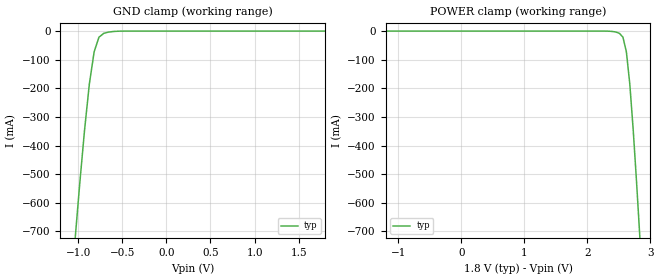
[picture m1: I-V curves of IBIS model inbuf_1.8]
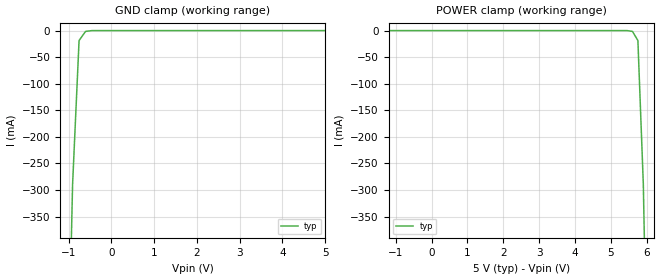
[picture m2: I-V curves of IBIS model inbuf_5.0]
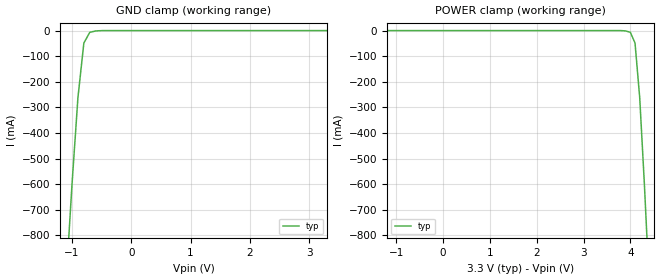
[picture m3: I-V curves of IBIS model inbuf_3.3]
|Texas Instruments Incorporated
|tmux2821, 2 Data Lane 1:1 15V Precision mux
[IBIS Ver]   4.1
[File name]   tmux2821.ibs
[Date]   04/10/25
[File Rev]   1.0
[Source]
| Texas Instruments Incorporated.
| ASC-INT-MPD
| 12500 TI Blvd
| Dallas, TX - 75243
[Notes]   Revision History:
| Rev 1.0: 04/10/25
| - Initial version of the model
| - Model generated from simulations in SPECTRE
| - C_comp although listed in numerical order of value are
|   obtained from varying PVT conditions. For PVT conditions for
|   each specific value refer the buffer description under
|   respective [Model]. IBIS model user is responsible for using
|   appropriate C_comp to simulate for Signal Integrity.
[Disclaimer]
| This model is designed as an aid for customers of Texas Instruments.
| TI and its licensors and suppliers make no warranties, either expressed
| or implied, with respect to this  model, including the warranties of
| merchantability or fitness for a particular purpose. The model is
| provided solely on an "as is" basis. The entire risk as to its quality
| and performance is with the customer.
| This model is subject to change without notice. Texas Instruments
| Incorporated is not responsible for updating this model.
[Copyright]
(C) Copyright 2025 Texas Instruments Incorporated.All rights reserved.
|  Component TMUX2821DSG 8-pin - DSG package
|  Part # TMUX2821DSG
[Component]   TMUX2821DSG
[Manufacturer]  TI
[Package]
|   typ   min   max
R_pkg   0.027   NA   NA
L_pkg   2.1992nH   NA   NA
C_pkg   0.2884pF   NA   NA
[Pin]   signal_name   model_name
   1   S1   sterm_fs_dual_7.5
   2   D1   dterm_fs_dual_7.5
   3   SEL2   inbuf
   4   GND   gnd
   5   S2   sterm_fs_dual_7.5
   6   D2   dterm_fs_dual_7.5
   7   SEL1   inbuf
   8   VDD   power
[Series Switch Groups]
On 1 /
On 2 /
Off 1 2 /
[Series Pin Mapping]  pin_2 model_name function_table_group
   1   2   switch_dual_7.5   1
   5   6   switch_dual_7.5   2
|  Component TMUX2821DDF 8-pin - DDF package
|  Part # TMUX2821DDF
[Component]   TMUX2821DDF
[Manufacturer]  TI
[Package]
|   typ   min   max
R_pkg   0.027   NA   NA
L_pkg   2.1992nH   NA   NA
C_pkg   0.2884pF   NA   NA
[Pin]   signal_name   model_name
   1   S1   sterm_fs_dual_7.5
   2   D1   dterm_fs_dual_7.5
   3   SEL2   inbuf
   4   GND   gnd
   5   S2   sterm_fs_dual_7.5
   6   D2   dterm_fs_dual_7.5
   7   SEL1   inbuf
   8   VDD   power
[Series Switch Groups]
On 1 /
On 2 /
Off 1 2 /
[Series Pin Mapping]  pin_2 model_name function_table_group
   1   2   switch_dual_7.5   1
   5   6   switch_dual_7.5   2
[Model Selector] inbuf
inbuf_1.8 Use for operation at 1V
inbuf_5.0 Use for operation at 5V
inbuf_3.3 Use for operation at 3V
| switch_dual_7.5
[Model]   switch_dual_7.5
Model_type   Series_switch
|   typ   min   max
C_comp   1.598234e-11   NA   NA
[Voltage Range]   7   NA   NA
[Power Clamp Reference]   0   NA   NA
[Temperature Range]   27   NA   NA
[On]
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[Off]
|   typ   min   max
[R Series]   10G   NA   NA
| Models and submodels in the file (6): inbuf_1.8 (Input), inbuf_5.0 (Input), inbuf_3.3 (Input), switch_dual_7.5 (Series_switch), dterm_fs_dual_7.5 (Terminator), sterm_fs_dual_7.5 (Terminator)
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| inbuf_1.8
[Model]   inbuf_1.8
Model_type   Input
Vinl = 0.549
Vinh = 0.589
|   typ   min   max
C_comp   2.533030e-12   NA   NA
[Voltage Range]   1.8   NA   NA
[Temperature Range]   27   NA   NA
[Power Clamp Reference]   1.8   NA   NA
[GND Clamp Reference]   0   NA   NA
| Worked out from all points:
|   GND clamp passes 1 mA (typ) near -0.58 V on its own axis
[GND Clamp]
|   Voltage   I(typ)   I(min)   I(max)
-3.6V     -6.952A    NA         NA
-1.036V   -735.7mA   NA         NA
-981.8mV  -534.4mA   NA         NA
-927.3mV  -347mA     NA         NA
-872.7mV  -185.3mA   NA         NA
-818.2mV  -72.18mA   NA         NA
-763.6mV  -21.27mA   NA         NA
-709.1mV  -7.922mA   NA         NA
-545.5mV  -422.6uA   NA         NA
1.8V      296.8nA    NA         NA
[POWER Clamp]
|   Voltage   I(typ)   I(min)   I(max)
-1.8V     593.7nA    NA         NA
2.291V    -92.86uA   NA         NA
2.4V      -1.377mA   NA         NA
2.509V    -7.922mA   NA         NA
2.564V    -21.27mA   NA         NA
2.618V    -72.18mA   NA         NA
2.673V    -185.3mA   NA         NA
2.727V    -347mA     NA         NA
2.782V    -534.4mA   NA         NA
2.836V    -735.7mA   NA         NA
3.6V      -3.295A    NA         NA
| inbuf_5.0
[Model]   inbuf_5.0
Model_type   Input
Vinl = 0.946
Vinh = 1.070
|   typ   min   max
C_comp   2.533030e-12   NA   NA
[Voltage Range]   5.0   NA   NA
[Temperature Range]   27   NA   NA
[Power Clamp Reference]   5.0   NA   NA
[GND Clamp Reference]   0   NA   NA
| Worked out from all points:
|   GND clamp passes 1 mA (typ) near -0.55 V on its own axis
[GND Clamp]
|   Voltage   I(typ)   I(min)   I(max)
-10V      -19.94A    NA         NA
-1.061V   -828.1mA   NA         NA
-909.1mV  -289.3mA   NA         NA
-757.6mV  -18.75mA   NA         NA
-606.1mV  -1.541mA   NA         NA
-454.5mV  -29.19uA   NA         NA
5V        824.6nA    NA         NA
[POWER Clamp]
|   Voltage   I(typ)   I(min)   I(max)
-5V       1.649uA    NA         NA
5.303V    -156.5nA   NA         NA
5.606V    -1.541mA   NA         NA
5.758V    -18.75mA   NA         NA
5.909V    -289.3mA   NA         NA
6.061V    -828.1mA   NA         NA
10V       -9.798A    NA         NA
| inbuf_3.3
[Model]   inbuf_3.3
Model_type   Input
Vinl = 0.790
Vinh = 0.869
|   typ   min   max
C_comp   2.533030e-12   NA   NA
[Voltage Range]   3.3   NA   NA
[Temperature Range]   27   NA   NA
[Power Clamp Reference]   3.3   NA   NA
[GND Clamp Reference]   0   NA   NA
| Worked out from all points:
|   GND clamp passes 1 mA (typ) near -0.57 V on its own axis
[GND Clamp]
|   Voltage   I(typ)   I(min)   I(max)
-6.6V     -13.05A    NA         NA
-1.1V     -980.8mA   NA         NA
-1V       -600.3mA   NA         NA
-900mV    -261.7mA   NA         NA
-800mV    -48.6mA    NA         NA
-700mV    -6.876mA   NA         NA
-500mV    -122.1uA   NA         NA
3.3V      544.2nA    NA         NA
[POWER Clamp]
|   Voltage   I(typ)   I(min)   I(max)
-3.3V     1.088uA    NA         NA
3.7V      -4.447uA   NA         NA
3.9V      -1.377mA   NA         NA
4V        -6.876mA   NA         NA
4.1V      -48.6mA    NA         NA
4.2V      -261.7mA   NA         NA
4.3V      -600.3mA   NA         NA
4.4V      -980.8mA   NA         NA
6.6V      -6.342A    NA         NA
